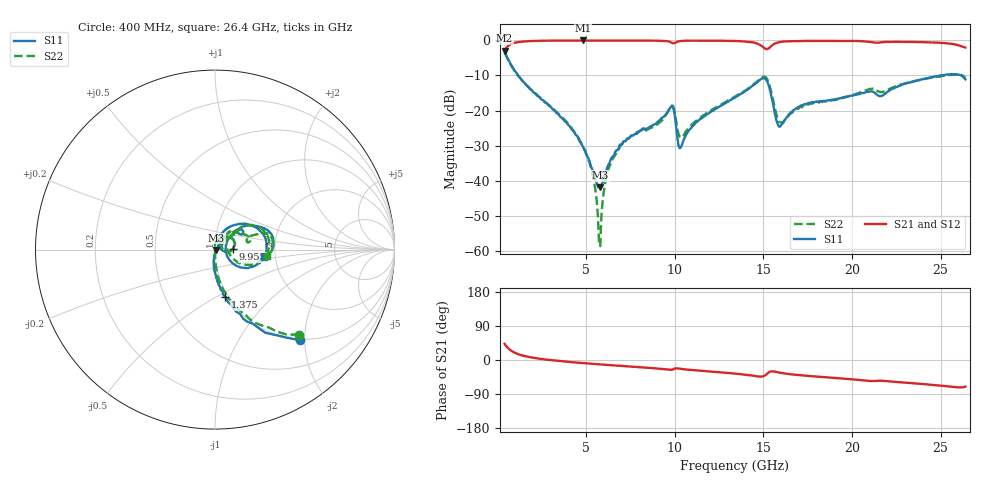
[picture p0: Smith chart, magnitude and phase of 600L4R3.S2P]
!  American Technical Ceramics  Date:  6/18/2004
!  One Norden Lane
!  Huntington Station,  NY.  11746-2102
!  Tel:  (631) 622-4700  Fax:  (631) 622-4748
!  Part Number  600L4R3  Mounting Orientation: Vertical
!  Description: Ultra Low ESR Microwave capacitors
!  Application: Coupling, Bypass, Tuning, DC Block
!  Filters, Matching
# GHZ S DB R 50
! Freq  |S11|  S11 Ph  |S21|  S21 Ph  |S12|  S12 Ph  |S22|  S22 Ph
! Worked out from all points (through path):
!   401 points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, 400 MHz to 26.4 GHz, reference 50 ohm
!   highest |S21| = -0.03 dB at 4.82 GHz (marker M1); lowest = -3.0 dB at 400 MHz (marker M2)
!   group delay of S21, straight-line fit = 8.6 ps
!   lowest |S11| = -41.9 dB at 5.795 GHz (marker M3), VSWR 1.02, Z = 50.8 - j0.198 ohm
!   |S11| at or under -10 dB: 1.154 GHz to 25 GHz (23.84 GHz wide, 182 % of centre); 26.17 GHz to end of sweep
!   |S22| runs from -58.6 to -3.5 dB; largest |S21 - S12| = 0.03
!   S11 on the Smith chart (normalised r, x): 400 MHz: 0.98, -1.91; 1.375 GHz: 0.97, -0.55; 9.955 GHz: 1.22, +0.01; 26.4 GHz: 1.75, -0.16
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0.4  -3.17 -46.7  -2.98 42.7  -3.26 43.9  -3.52 -45.3
1.375  -11.40 -77.5  -0.36 12.2  -0.38 13.4  -11.35 -75.1
4.755  -29.71 -95.9  -0.03 -7.9  0.00 -7.9  -29.64 -88.0
4.82  -30.40 -94.5  -0.03 -8.2  0.00 -8.2  -30.25 -89.0
5.34  -36.58 -80.0  -0.03 -10.1  -0.02 -10.1  -37.65 -89.8
5.535  -39.79 -61.8  -0.03 -10.7  -0.01 -10.7  -43.07 -93.0
5.665  -41.78 -40.8  -0.03 -11.2  -0.03 -11.2  -50.09 -98.9
5.795  -41.86 -13.9  -0.03 -11.6  -0.03 -11.6  -58.63 131.9
6.12  -37.44 27.6  -0.04 -12.8  -0.04 -12.6  -39.49 93.8
6.64  -31.72 40.8  -0.05 -14.5  -0.02 -13.9  -32.76 90.3
7.615  -27.14 49.3  -0.05 -17.6  -0.01 -17.7  -27.01 85.3
9.11  -22.89 57.0  -0.12 -22.9  -0.09 -23.1  -23.53 65.0
9.76  -19.04 35.8  -0.50 -26.1  -0.48 -26.2  -18.99 37.5
9.955  -19.93 2.3  -0.84 -23.5  -0.81 -23.8  -19.47 3.3
10.345  -30.47 40.1  -0.18 -23.4  -0.16 -23.7  -27.75 16.6
11.255  -23.24 69.3  -0.07 -27.5  -0.07 -27.7  -22.71 40.9
13.4  -16.30 56.4  -0.20 -35.8  -0.19 -35.8  -16.00 41.3
15.09  -10.86 -2.1  -2.32 -40.9  -2.31 -41.1  -10.37 3.5
15.935  -24.58 3.9  -0.48 -33.6  -0.49 -34.0  -23.31 4.8
17.755  -17.59 39.3  -0.16 -42.9  -0.24 -42.8  -18.07 50.2
22.11  -14.25 40.8  -0.41 -56.4  -0.41 -56.2  -13.88 20.7
26.4  -11.12 -8.5  -2.04 -70.2  -2.03 -70.3  -10.71 -6.9
